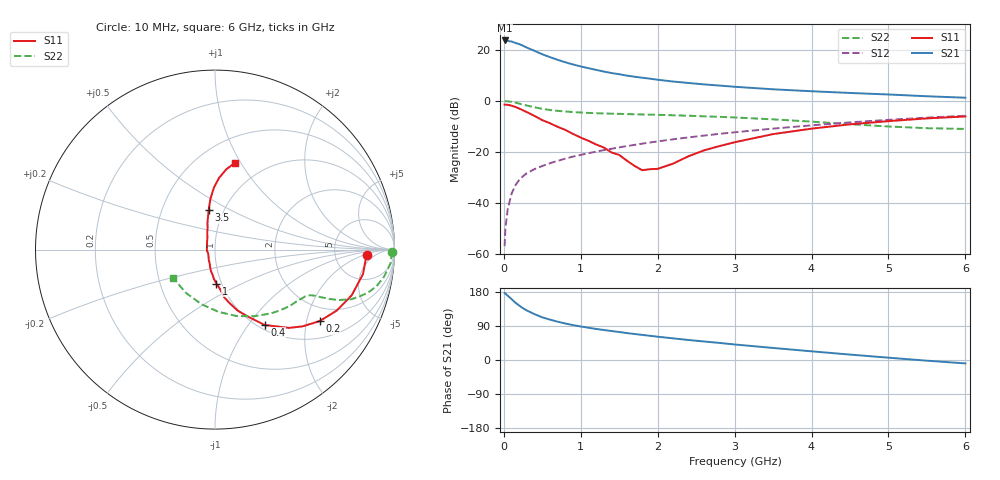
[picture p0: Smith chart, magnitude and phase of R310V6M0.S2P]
! SIEMENS Small Signal Semiconductors
! BFR181
! Si NPN RF Bipolar Junction Transistor in SOT23
! VCE = 10 V  IC = 6 mA
! Common Emitter S-Parameters:  May  1996
# GHz  S  MA  R  50
!  f  S11  S21  S12  S22
! GHz  MAG  ANG  MAG  ANG  MAG  ANG  MAG  ANG
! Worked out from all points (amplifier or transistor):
!   36 points, 10 MHz to 6 GHz, reference 50 ohm
!   highest |S21| = 23.7 dB at 10 MHz (marker M1)
!   |S21| within 3 dB of that: start of sweep to 314.2 MHz
!   unconditionally stable (mu >= 1): 1.136 GHz to 3.083 GHz
!   at 250 MHz: K = 0.46, MSG = 25.6 dB, |S12| = -29.6 dB
!   at 1.4 GHz: K = 1.04, MAG = 13.7 dB, |S12| = -18.8 dB
!   at 6 GHz: K = 0.87, MSG = 3.5 dB, |S12| = -5.8 dB
!   S11 on the Smith chart (normalised r, x): 10 MHz: 11, -2; 200 MHz: 1.51, -2.39; 400 MHz: 1.07, -1.21; 1 GHz: 0.95, -0.37; 3.5 GHz: 0.85, +0.39; 6 GHz: 0.74, +0.94
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0.01  0.8446 -1.9  15.35 176.9  0.0014 91.5  0.9885 -0.8
0.02  0.8413 -3.8  14.91 175.1  0.0031 84.7  0.9853 -1.9
0.05  0.8358 -9.4  15.02 169.8  0.0074 86.4  0.9799 -4.6
0.1  0.8031 -18.5  14.64 160.7  0.015 80.0  0.9546 -9.0
0.15  0.758 -26.7  13.73 151.3  0.022 75.8  0.9229 -12.8
0.2  0.7058 -34.4  13.02 143.6  0.0281 72.1  0.8831 -15.9
0.25  0.649 -41.2  12.08 136.5  0.0331 69.3  0.8418 -18.2
0.3  0.6014 -46.5  11.1 130.6  0.0381 68.0  0.8081 -20.0
0.4  0.5042 -56.5  9.581 120.9  0.0457 66.4  0.7464 -22.1
0.5  0.418 -63.6  8.219 112.5  0.0526 65.3  0.6962 -23.3
0.6  0.363 -69.6  7.213 106.5  0.0597 64.8  0.6617 -23.9
0.8  0.2685 -79.3  5.712 96.3  0.0734 64.9  0.6179 -24.7
1  0.1901 -87.5  4.742 88.4  0.0869 65.4  0.5902 -25.5
1.1  0.1642 -91.9  4.38 85.2  0.0938 65.4  0.5797 -26.1
1.3  0.1214 -100.7  3.761 79.2  0.1078 65.4  0.5655 -27.5
1.6  0.0667 -121.2  3.131 71.0  0.1294 64.7  0.5501 -30.1
1.8  0.0434 -152.4  2.842 66.2  0.1446 64.2  0.5399 -32.1
2.2  0.0585 139.4  2.395 57.1  0.1755 62.5  0.5217 -37.0
3.5  0.2223 99.2  1.686 31.8  0.285 53.0  0.4328 -58.9
4.5  0.3458 91.0  1.429 14.3  0.378 43.0  0.3478 -86.6
5.5  0.4526 81.9  1.231 -1.8  0.4682 31.0  0.2904 -124.1
6  0.4941 77.2  1.153 -9.0  0.5105 24.3  0.2809 -145.4
